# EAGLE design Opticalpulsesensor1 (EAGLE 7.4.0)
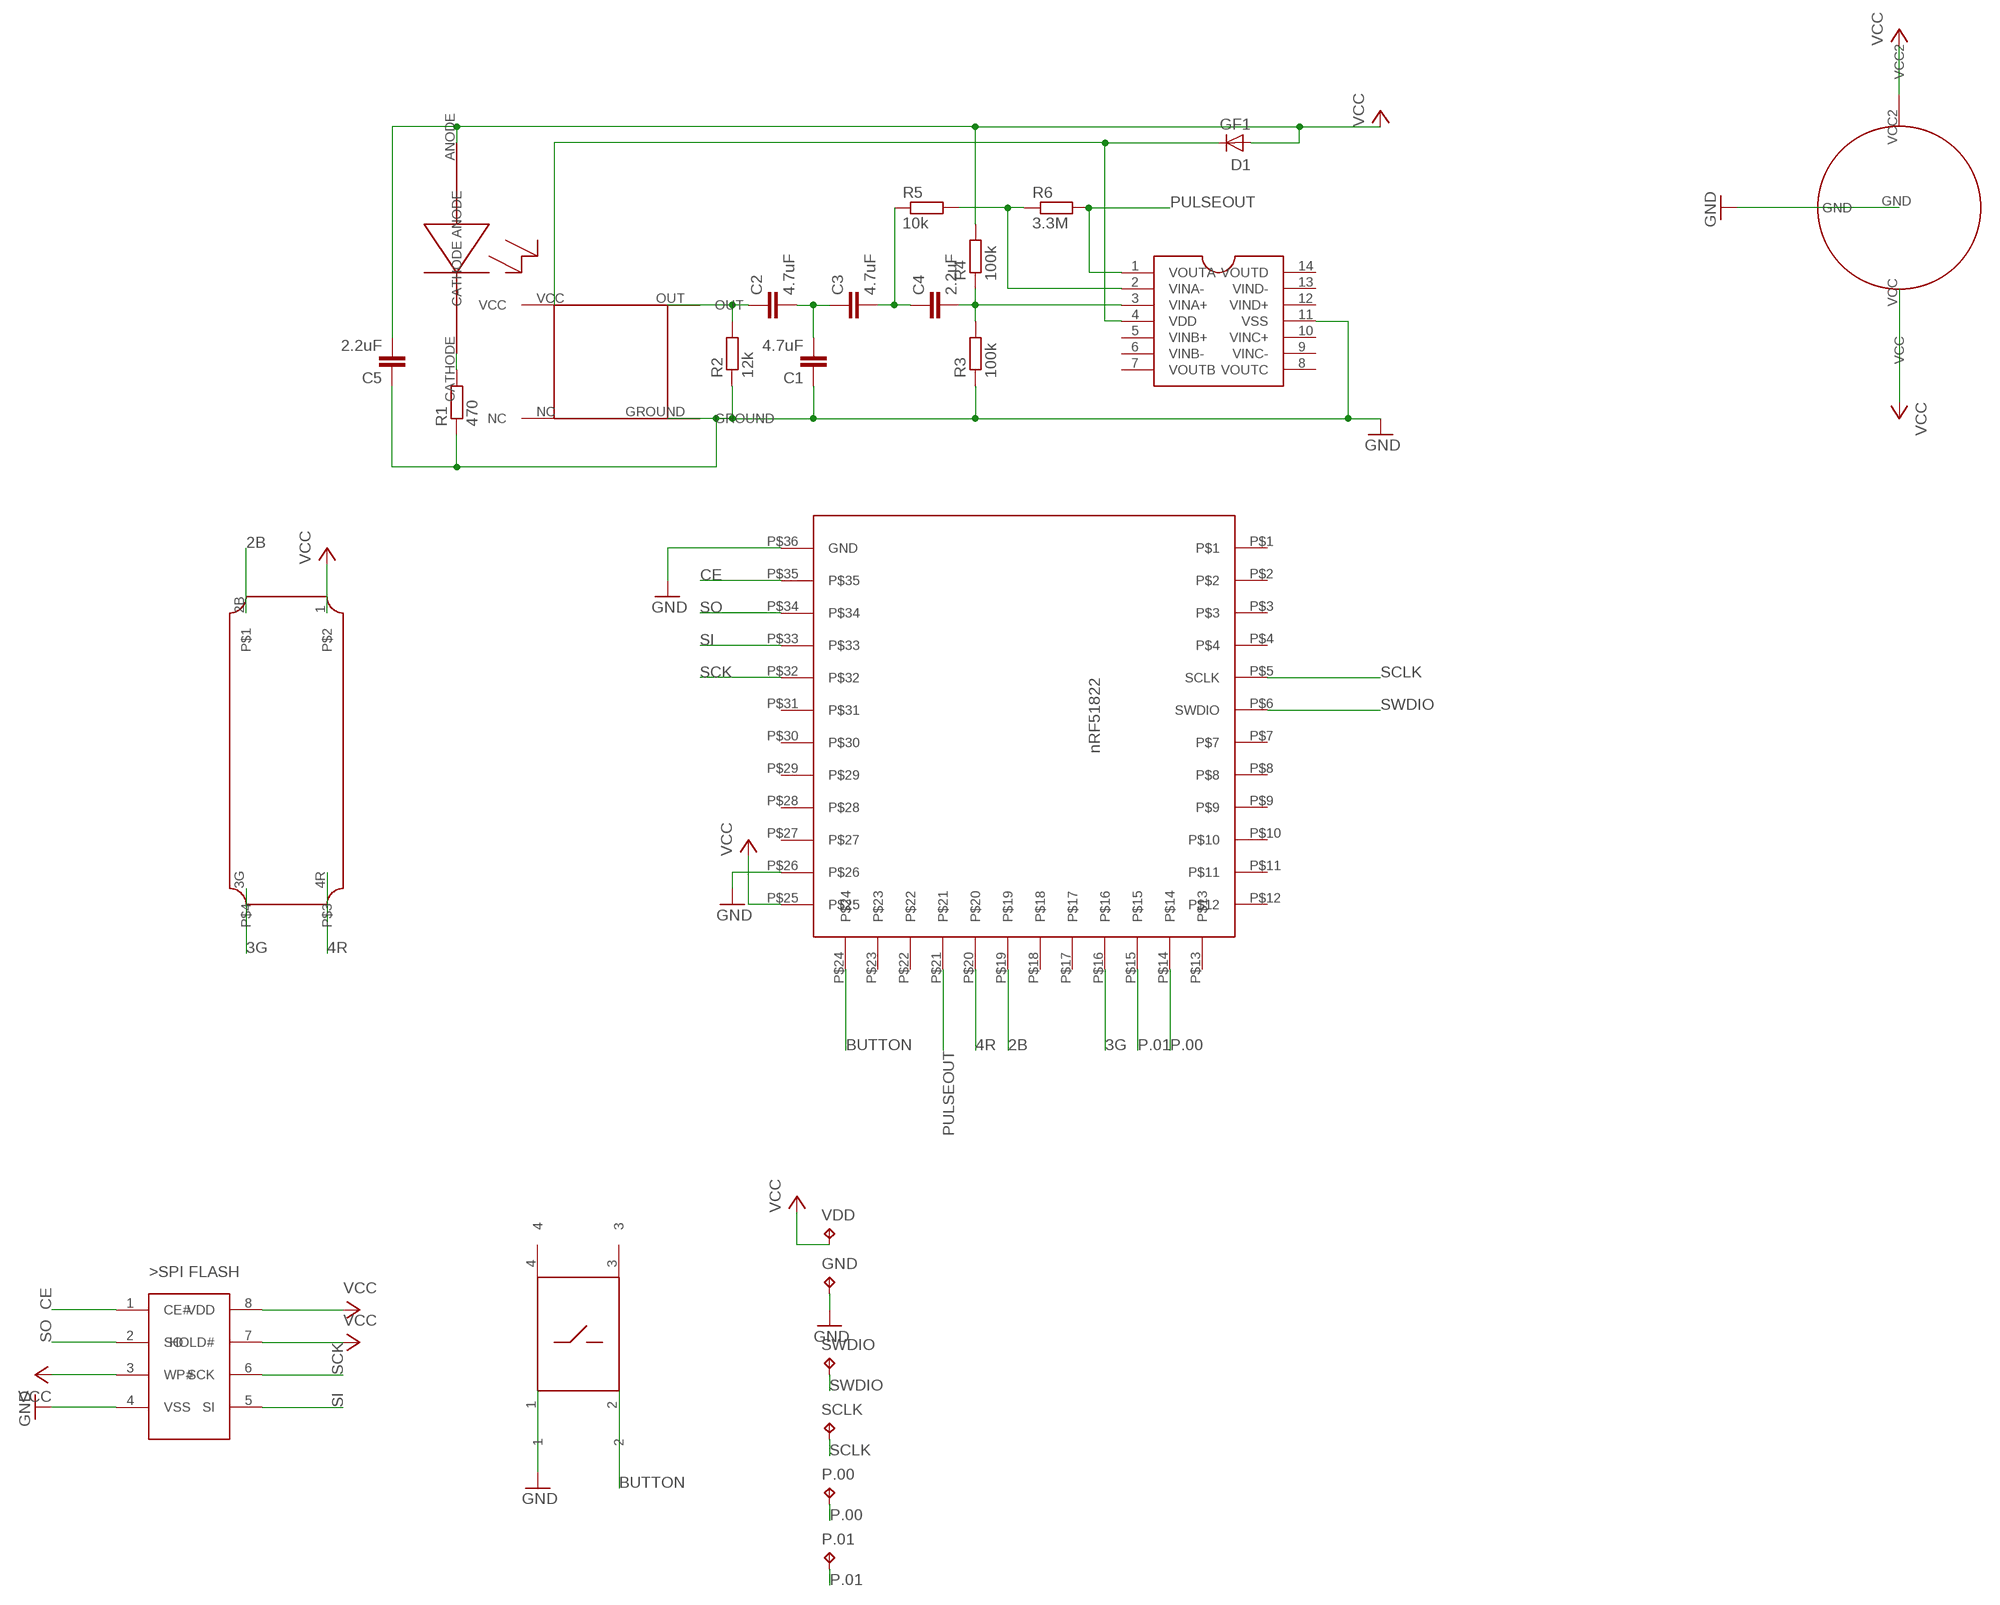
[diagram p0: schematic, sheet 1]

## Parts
C1  4.7uF  C-EUC0805  [C0805]
C2  4.7uF  C-EUC0805  [C0805]
C3  4.7uF  C-EUC0805  [C0805]
C4  2.2uF  C-EUC0805  [C0805]
C5  2.2uF  C-EUC0805  [C0805]
D1  GF1  [SMA-DO214AC]
GND  TPTP09SQ  [TP09SQ]
P.00  TPTP09SQ  [TP09SQ]
P.01  TPTP09SQ  [TP09SQ]
R1  470  R-EU_M0805  [M0805]
R2  12k  R-EU_M0805  [M0805]
R3  100k  R-EU_M0805  [M0805]
R4  100k  R-EU_M0805  [M0805]
R5  10k  R-EU_M0805  [M0805]
R6  3.3M  R-EU_M0805  [M0805]
SCLK  TPTP09SQ  [TP09SQ]
SWDIO  TPTP09SQ  [TP09SQ]
U$1  LIGHTSENSOR  [LIGHTSENSOR]
U$2  OPAMP  [TSSOP-14]
U$3  GREENLED  [GREENLED]
U$4  BATTERY  [BATTERY]
U$5  NRF51822  [NRF51822]
U$6  BUTTON1  [BUTTON1]
U$7  RGB  [RGB]
U$8  SPI_FLASH  [SOIC-8]
VDD  TPTP09SQ  [TP09SQ]

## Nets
2B: U$5.P$19 U$7.2B
3G: U$5.P$16 U$7.3G
4R: U$5.P$20
BUTTON: U$5.P$24 U$6.2
CE: U$5.P$35 U$8.1(CE#)
GND: C1.1 C5.1 GND.TP R1.1 R2.1 R3.1 U$1.GROUND U$2.11(VSS) U$4.GND U$5.P$26 U$5.P$36(GND) U$6.1 U$8.4(VSS)
N$2: C4.2 R3.2 R4.1 U$2.3(VINA+)
N$3: C3.2 C4.1 R5.1
N$4: D1.K(C) U$1.VCC U$2.4(VDD)
N$7: R5.2 R6.1 U$2.2(VINA-)
N$8: C1.2 C2.2 C3.1
N$9: C2.1 R2.2 U$1.OUT
N$10: R1.2 U$3.CATHODE
P.00: P.00.TP U$5.P$14
P.01: P.01.TP U$5.P$15
PULSEOUT: R6.2 U$2.1(VOUTA) U$5.P$21
SCK: U$5.P$32 U$8.6(SCK)
SCLK: SCLK.TP U$5.P$5(SCLK)
SI: U$5.P$33 U$8.5(SI)
SO: U$5.P$34 U$8.2(SO)
SWDIO: SWDIO.TP U$5.P$6(SWDIO)
VCC: C5.2 D1.A R4.2 U$3.ANODE U$4.VCC U$5.P$25 U$7.1 U$8.3(WP#) U$8.7(HOLD#) U$8.8(VDD) VDD.TP
Unconnected: U$1.NC U$2.5(VINB+) U$2.6(VINB-) U$2.7(VOUTB) U$2.8(VOUTC) U$2.9(VINC-) U$2.10(VINC+) U$2.12(VIND+) U$2.13(VIND-) U$2.14(VOUTD) U$4.VCC2 U$5.P$1 U$5.P$2 U$5.P$3 U$5.P$4 U$5.P$7 U$5.P$8 U$5.P$9 U$5.P$10 U$5.P$11 U$5.P$12 U$5.P$13 U$5.P$17 U$5.P$18 U$5.P$22 U$5.P$23 U$5.P$27 U$5.P$28 U$5.P$29 U$5.P$30 U$5.P$31 U$6.3 U$6.4 U$7.4R

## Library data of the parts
C1-C5 = rcl:C-EU: CAPACITOR, European symbol
D1 = diode:GF1: DIODE
GND P.00 P.01 SCLK SWDIO VDD = testpad:TP: Test pad
R1-R6 = rcl:R-EU_: RESISTOR, European symbol
U$1 = lightsensor:LIGHTSENSOR
U$2 = soic8:OPAMP
U$3 = GREENLED:GREENLED
U$4 = bat:BATTERY
U$5 = nrf51822:NRF51822
U$6 = button1:BUTTON1
U$7 = rgb:RGB
U$8 = soic8:SPI_FLASH

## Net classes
0 default: width 0.4 mm, drill 0.254 mm, clearance 0.254 mm

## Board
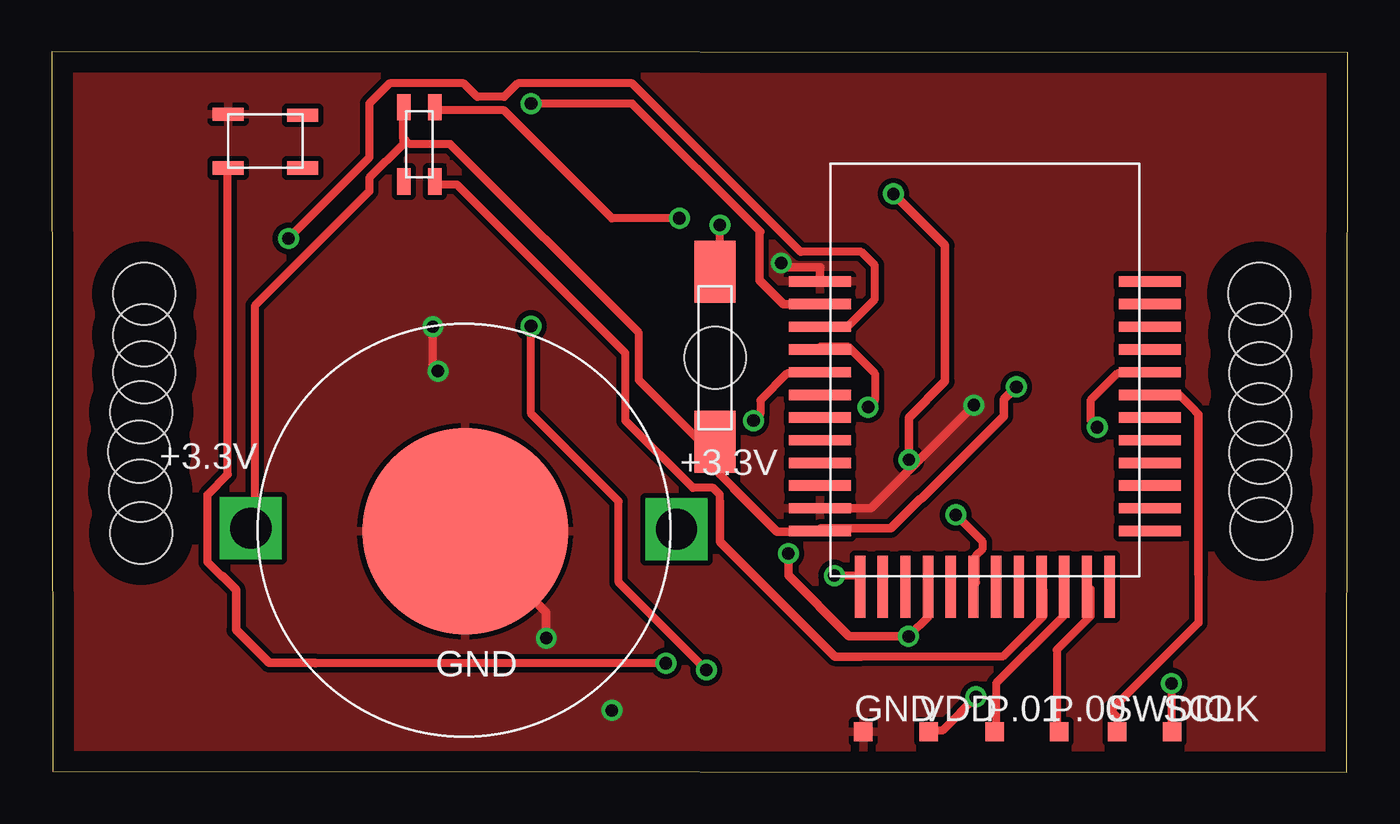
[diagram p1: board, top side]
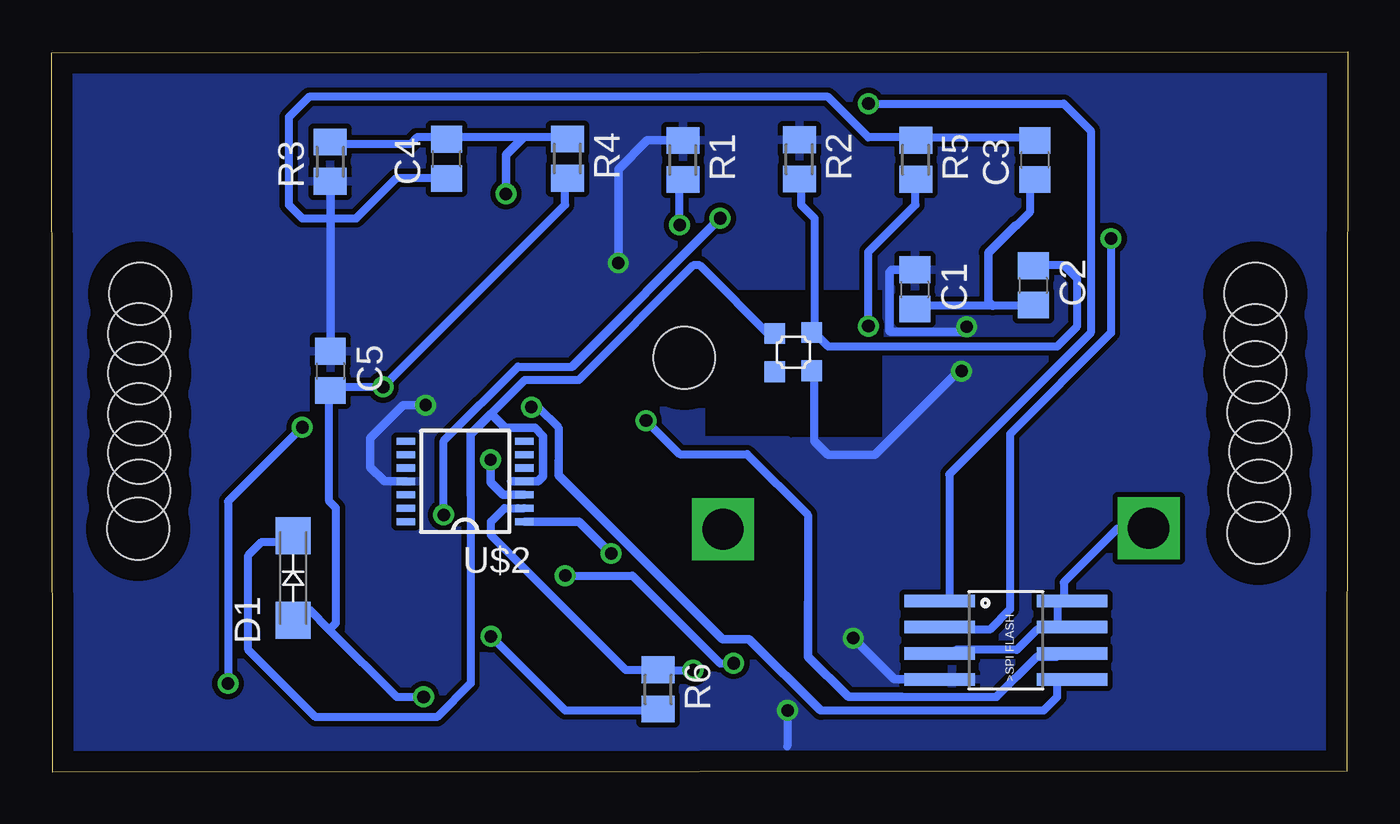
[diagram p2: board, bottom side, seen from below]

Size 62.9 x 34.95 mm. Coordinates in mm from the lower left corner, seen from the top.
Outline: 0.05,0.05 62.85,0 62.9,34.9 0,34.95 0.05,0.05
Copper layers (1*16): Top 0.035mm / dielectric 1.5mm / Bottom 0.035mm
Design rules "default *": minimum track width 10mil, minimum drill 24mil, track to track 10mil, track to pad 10mil, pad to pad 10mil, via to via 10mil, smd to smd 10mil, copper to edge 40mil, drill to drill 10mil, minimum pad ring 10mil, minimum via ring 8mil, stop-mask expansion 4mil, vias tented up to drill 0mil, thermal gap 10mil
Holes 3 mm at 32.2,20.1 4.5,23.2 4.5,21.2 4.5,19.4 4.35,17.45 4.25,15.55 4.3,13.65 4.35,11.6 58.6,23.2 58.65,21.25 58.65,19.35 58.65,17.35 58.65,15.5 58.65,13.65 58.7,11.8

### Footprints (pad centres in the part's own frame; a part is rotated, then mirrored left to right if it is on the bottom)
C0805 = smd 1.3 x 1.5: 1 -0.95,0; 2 0.95,0
SMA-DO214AC = smd 1.8 x 1.7: A -2.05,0; K 2.05,0
TP09SQ = smd 0.9 x 0.9: TP 0,0
M0805 = smd 1.3 x 1.6: 1 -0.95,0; 2 0.95,0
LIGHTSENSOR = smd 1 x 1: GROUND -0.15,-0.1; NC -0.2,1.7; OUT 1.7,-0.1; VCC 1.65,1.7
TSSOP-14 = smd 0.9 x 0.35: 1 -2.875,1.95; 2 -2.875,1.3; 3 -2.875,0.65; 4 -2.875,0; 5 -2.875,-0.65; 6 -2.875,-1.3; 7 -2.875,-1.95; 8 2.875,-1.95; 9 2.875,-1.3; 10 2.875,-0.65; 11 2.875,0; 12 2.875,0.65; 13 2.875,1.3; 14 2.875,1.95
GREENLED = smd 3 x 2: ANODE -0.6,0.8; CATHODE 7.65,0.8
BATTERY = smd 10 x 10: GND 0.05,-0.05 | drill 2 square: VCC -10.35,0.1; VCC2 10.3,0.05
NRF51822 = smd 0.5 x 3: P$1 -4.3,8; P$2 -3.2,8; P$3 -2.1,8; P$4 -1,8; P$5 0.1,8; P$6 1.2,8; P$7 2.3,8; P$8 3.4,8; P$9 4.5,8; P$10 5.6,8; P$11 6.7,8; P$12 7.8,8; P$25 7.8,-8; P$26 6.7,-8; P$27 5.6,-8; P$28 4.5,-8; P$29 3.4,-8; P$30 2.3,-8; P$31 1.2,-8; P$32 0.1,-8; P$33 -1,-8; P$34 -2.1,-8; P$35 -3.2,-8; P$36 -4.3,-8 | smd 3 x 0.5: P$13 10.5,6.05; P$14 10.5,4.95; P$15 10.5,3.85; P$16 10.5,2.75; P$17 10.5,1.65; P$18 10.5,0.55; P$19 10.5,-0.55; P$20 10.5,-1.65; P$21 10.5,-2.75; P$22 10.5,-3.85; P$23 10.5,-4.95; P$24 10.5,-6.05
BUTTON1 = smd 1.5 x 0.65: 1 0,2.6; 2 0,0; 3 3.6,0; 4 3.6,2.55
RGB = smd 1.27 x 0.66: 1 -0.2,-0.1; 2B -0.2,1.4; 3G 3.4,1.4; 4R 3.4,-0.1
SOIC-8 = smd 0.61 x 2.21: 1 -1.905,-2.616; 2 -0.635,-2.616; 3 0.635,-2.616; 4 1.905,-2.616; 5 1.905,2.616; 6 0.635,2.616; 7 -0.635,2.616; 8 -1.905,2.616 | smd 0.609 x 0.609: P$1 -1.904,4.015; P$2 -1.904,4.612; P$3 -0.636,4.015; P$4 -0.636,4.616; P$5 0.636,4.015; P$6 0.636,4.62; P$7 1.904,4.022; P$8 1.904,4.629; P$9 -1.902,-4.016; P$10 -1.902,-4.615; P$11 -0.636,-4.016; P$12 -0.636,-4.621; P$13 0.636,-4.016; P$14 0.636,-4.621; P$15 1.902,-4.016; P$16 1.902,-4.621

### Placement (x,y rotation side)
C1  21.02,23.41 270 bottom
C2  15.27,23.61 270 bottom
C3  15.18,29.69 90 bottom
C4  43.73,29.74 90 bottom
C5  49.37,19.46 270 bottom
D1  51.18,9.41 90 bottom
GND  39.39,1.96 0 top
P.00  48.88,1.96 0 top
P.01  45.75,1.96 0 top
R1  32.27,29.69 270 bottom
R2  26.62,29.72 270 bottom
R3  49.38,29.61 90 bottom
R4  37.87,29.76 270 bottom
R5  20.97,29.7 270 bottom
R6  33.47,4.01 270 bottom
SCLK  54.37,1.96 0 top
SWDIO  51.7,1.96 0 top
U$1  26.11,19.62 90 bottom
U$2  42.83,14.1 180 bottom
U$3  32.99,16.62 90 top
U$4  20.02,11.73 0 top
U$5  45.28,19.5 270 top
U$6  8.58,29.31 0 top
U$7  17.2,32.05 270 top
U$8  16.6,6.4 270 bottom
VDD  42.56,1.96 0 top

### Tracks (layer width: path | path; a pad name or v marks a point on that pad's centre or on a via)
2B  (via drill 0.61)
  Top 0.4: v30.46,26.86 27.19,26.86 21.96,32.1 18.69,32.1 U$7.2B | v43.87,12.48 45.18,11.17 45.18,10.84 44.85,10.51 44.85,9.21 U$5.P$19
  Bottom 0.4: 37.65,19.67 40.27,19.67 43.87,16.07 v43.87,12.48
  Bottom 0.406: v30.46,26.86 37.65,19.67
3G
  Top 0.4: 32.42,13.13 32.42,13.46 32.1,13.78 31.12,13.78 27.85,17.05 27.85,20.32 19.67,28.5 18.69,28.5 U$7.3G | 39.29,5.61 46.16,5.61 48.12,7.57 48.12,8.88 U$5.P$16
  Top 0.406: 32.42,13.13 32.42,11.18 38,5.6 39.28,5.6 39.29,5.61
BUTTON  (via drill 0.61)
  Top 0.4: 8.23,9.53 7.57,10.19 7.57,13.46 8.55,14.44 8.55,29.15 U$6.2 | v29.81,5.28 12.8,5.28 | v37.98,9.53 39.29,9.53 39.29,9.21 U$5.P$24
  Top 0.406: 8.23,9.53 8.27,9.53 8.95,8.85 8.95,6.9 10.55,5.3 12.79,5.3 12.8,5.28
  Bottom 0.4: v29.81,5.28 30.46,5.28 34.71,9.53 v37.98,9.53
CE  (via drill 0.61)
  Top 0.4: v23.27,32.42 28.17,32.42 34.38,26.21
  Top 0.406: U$5.P$35 35.5,22.7 34.35,23.85 34.35,26.18 34.38,26.21
  Bottom 0.4: v23.27,32.42 13.78,32.42 12.48,31.12 12.48,21.3 19.34,14.44 19.34,8.55 U$8.1
GND  (via drill 0.6, 0.61)
  Top 0.406: v24,6.5 24,7.75 U$4.GND | U$5.P$36 37.28,24.48 37.3,24.5 35.6,24.5 v35.4,24.7 | U$5.P$26 39.75,12.8 v44.75,17.8 | v18.5,21.6 18.5,19.7 v18.75,19.45
  Bottom 0.4: 25.88,16.05 25.88,19.34 U$1.GROUND | v27.19,2.99 27.2,1.25
  Bottom 0.406: U$8.4 22,4.5 v24,6.5 | v35.4,24.7 35.4,29.25 34,30.65 R1.1 | C5.1 R3.1 | v44.75,17.8 45.85,17.8 47.45,16.2 47.45,14.8 46.75,14.1 U$2.11 | C1.1 22.14,24.36 22.25,24.25 22.25,21.4 22.2,21.35 18.75,21.35 v18.5,21.6 | v18.75,19.45 18.9,19.45 22.95,15.4 25.23,15.4 25.88,16.05
  pour Top: -0.05,34.95 62.9,34.95 62.9,0.05 -0.05,0.05
  pour Bottom: 0.05,34.85 62.85,34.85 62.85,0.05 27.2,0.05 27.2,16.1 31.4,16.1 31.4,23.6 22.4,23.6 22.4,16.05 26.9,16.05 26.9,0 0.05,0
N$2  (via drill 0.6)
  Top 0.406: v41.6,15.15 41.6,17.2 43.35,18.95 43.35,25.55 v40.85,28.05
  Bottom 0.4: R4.1 37.98,30.79 40,30.79 43.54,30.79 C4.2 43.87,30.79 45.18,30.79 45.5,30.46 49.1,30.46 R3.2
  Bottom 0.406: 40.85,13.45 U$2.3 41,13.45 41.6,14.05 v41.6,15.15 | v40.85,28.05 40.85,29.94 40,30.79
N$3
  Bottom 0.4: C3.2 15.42,30.79 20.65,30.79 R5.1 20.98,30.79 23.27,30.79 25.23,32.75 50.41,32.75 51.39,31.77 51.39,27.52 50.73,26.86 48.12,26.86 46.16,28.83 43.87,28.83 C4.1
N$4
  Bottom 0.4: 40.6,14.11 40.27,14.11 U$2.4 | 41.58,17.38 39.94,19.02 37.33,19.02 31.77,24.57 31.44,24.57 27.85,20.98 U$1.VCC | 42.56,13.46 42.56,4.3 44.2,2.67 50.08,2.67 53.35,5.94 53.35,10.51 52.7,11.17 51.39,11.17 D1.K
  Bottom 0.406: 40.6,14.11 39.29,14.11 39.05,14.35 39.05,16.3 39.45,16.7 40.9,16.7 41.58,17.38 42.56,16.4 42.56,13.46
N$7  (via drill 0.61)
  Top 0.4: v23.27,21.63 23.27,17.38 27.52,13.13 27.52,9.21 v31.77,4.96
  Bottom 0.4: U$2.2 40.27,12.8 40.92,12.8 41.58,12.15 41.58,11.5 35.04,4.96 33.73,4.96 R6.1 33.4,4.96 v31.77,4.96 | v23.27,21.63 23.27,25.23 20.98,27.52 20.98,28.5 R5.2
N$8
  Bottom 0.254: 15.3,22.55 C2.2
  Bottom 0.4: C1.2 20.98,22.61 17.25,22.61 15.42,22.61 C2.2 | 16.07,26.54 15.42,27.19 15.42,28.5 C3.1
  Bottom 0.406: 15.3,22.55 15.3,22.45 | 16.07,26.54 16.11,26.54 17.45,25.2 17.45,22.81 17.25,22.61
N$9
  Bottom 0.4: R2.2 26.54,28.5 26.54,27.52 25.88,26.86 25.88,21.63 U$1.OUT 25.88,21.3 25.23,20.65 14.11,20.65 13.13,21.63 13.13,23.92 13.78,24.57 15.09,24.57 C2.1
N$10  (via drill 0.61)
  Top 0.4: v32.42,26.54 32.42,24.57 U$3.CATHODE
  Bottom 0.4: v32.42,26.54 32.42,28.5 R1.2
P.00
  Top 0.4: P.00.TP 48.77,2.01 48.77,5.94 50.41,7.57 50.41,8.88 U$5.P$14
P.01
  Top 0.4: P.01.TP 45.83,2.01 45.83,4.3 49.1,7.57 49.1,8.88 U$5.P$15
PULSEOUT  (via drill 0.6, 0.61)
  Top 0.4: v41.58,6.59 42.56,7.57 42.56,8.88 U$5.P$21
  Top 0.406: v35.75,10.6 35.75,9.55 38.7,6.6 41.57,6.6 v41.58,6.59
  Bottom 0.4: v41.58,6.59 37.98,2.99 33.73,2.99 R6.2
  Bottom 0.406: U$2.1 37.3,12.15 v35.75,10.6
SCK  (via drill 0.61)
  Top 0.4: v34.06,17.05 34.38,17.38 34.38,18.04 35.69,19.34 37,19.34 U$5.P$32
  Bottom 0.4: 21.63,3.65 17.05,3.65 15.09,5.61 14.11,5.61 U$8.6 | 26.21,8.23 26.21,12.48 29.15,15.42 32.42,15.42 v34.06,17.05
  Bottom 0.406: 21.63,3.65 24.25,3.65 26.2,5.6 26.2,8.21 26.21,8.23
SCLK  (via drill 0.61)
  Top 0.4: v54.33,4.3 54.33,2.01 SCLK.TP | v50.73,16.73 50.41,17.05 50.41,18.04 51.72,19.34 53.02,19.34 U$5.P$5
  Bottom 0.4: v54.33,4.3 54.33,13.13 v50.73,16.73
SI  (via drill 0.61)
  Top 0.4: v39.62,17.71 39.94,18.04 39.94,19.34 38.64,20.65 37.33,20.65 U$5.P$33
  Bottom 0.4: 25.56,2.99 14.77,2.99 14.11,3.65 14.11,4.3 U$8.5 | 38.31,15.09 38.31,16.73 39.29,17.71 v39.62,17.71
  Bottom 0.406: 38.31,15.09 38.31,14.41 30.35,6.45 29.05,6.45 25.59,2.99 25.56,2.99
SO  (via drill 0.61)
  Top 0.4: v11.5,25.88 15.42,29.81 15.42,32.42 16.4,33.4 20,33.4 20.65,32.75 21.96,32.75 22.61,33.4 28.17,33.4 36.35,25.23 39.29,25.23 39.94,24.57 39.94,22.94 38.64,21.63 37.33,21.63 U$5.P$34
  Bottom 0.4: v11.5,25.88 11.5,21.3 16.4,16.4 16.4,7.9 17.38,6.92 19.02,6.92 U$8.2
SWDIO
  Top 0.4: 55.64,10.51 55.64,9.6 55.64,7.24 51.39,2.99 51.72,2.67 51.72,2.01 SWDIO.TP | 55.31,17.71 54.66,18.36 53.35,18.36 U$5.P$6
  Top 0.406: 55.31,17.71 55.31,17.69 55.65,17.35 55.65,9.61 55.64,9.6
VCC  (via drill 0.61)
  Top 0.4: v44.85,3.65 43.21,2.01 42.56,2.01 VDD.TP | 17.05,30.79 17.05,32.1 U$7.1 | 17.05,30.79 17.38,30.46 19.34,30.46 28.5,21.3 28.5,19.02 31.44,16.07 32.1,16.07 U$3.ANODE 32.42,15.75 32.42,14.44 33.08,13.78 | 17.05,30.79 17.05,30.46 15.42,28.83 15.42,28.17 9.86,22.61 9.86,12.15 U$4.VCC | 37.33,11.82 U$5.P$25
  Top 0.406: 37.33,11.82 40.72,11.82 42.15,13.25 42.2,13.25 46.2,17.25 46.2,18.08 v46.81,18.69 | 33.08,13.78 33.08,13.77 35.2,11.65 37.23,11.65 U$5.P$25
  Bottom 0.4: v44.85,3.65 46.16,3.65 49.43,6.92 | 49.43,6.92 50.41,7.9 50.73,7.9 51.06,7.57 D1.A | 49.43,6.92 49.1,7.24 49.1,12.8 49.43,13.13 49.43,18.36 C5.2 49.1,18.69 v46.81,18.69 37.98,27.52 37.98,28.5 R4.2 | U$8.3 19.02,5.94 16.07,5.94 15.09,6.92 14.11,6.92 U$8.7 14.11,7.24 14.11,8.23 U$8.8 13.78,8.55 13.78,9.21 11.17,11.82 9.86,11.82 U$4.VCC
